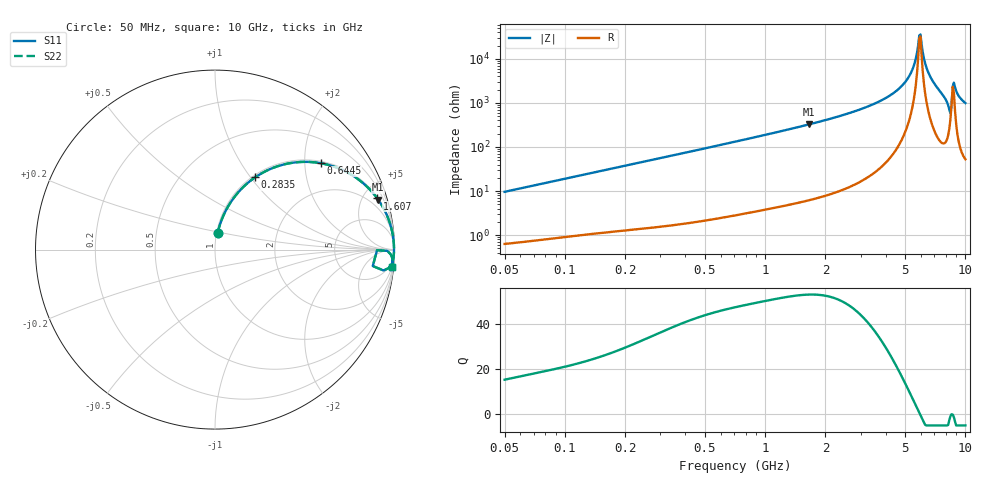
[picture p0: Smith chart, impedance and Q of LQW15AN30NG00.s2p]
!Murata Part Number: LQW15AN30NG00
!These Parameters are Measured in Series Mode Connection
!  o--[Z]--o
!Port1  Port2
!  o-------o
!Freq. Start=50[MHz] Stop=10[GHz], 401[Steps]
# Hz S RI R 50
!Freq.(Hz)	S 11(Real)	S 11(Imag)	S 21(Real)	S 21(Imag)	S 12(Real)	S 12(Imag)	S 22(Real)	S 22(Imag)
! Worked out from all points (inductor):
!   401 points, 50 MHz to 10 GHz, reference 50 ohm
!   read as one part in series: L = 30.3 nH near 51.34 MHz
!   highest Q = 52.9 at 1.651 GHz (marker M1), where L = 31.3 nH
!   self-resonance near 5.887 GHz
!   S11 on the Smith chart (normalised r, x): 50 MHz: 1.01, +0.19; 283.5 MHz: 1.03, +1.05; 644.5 MHz: 1.05, +2.40; 1.607 GHz: 1.12, +6.30; 10 GHz: 2, -20
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5e7  0.0151 0.0936  0.9849 -0.0936  0.9849 -0.0936  0.0151 0.0936
1.214486e8  0.0581 0.2131  0.9419 -0.2131  0.9419 -0.2131  0.0581 0.2131
2.835028e8  0.2239 0.4029  0.7761 -0.4029  0.7761 -0.4029  0.2239 0.4029
2.949953e8  0.2373 0.4117  0.7627 -0.4117  0.7627 -0.4117  0.2373 0.4117
6.444912e8  0.5879 0.4816  0.4121 -0.4816  0.4121 -0.4816  0.5879 0.4816
7.071068e8  0.6317 0.4719  0.3683 -0.4719  0.3683 -0.4719  0.6317 0.4719
1.607477e9  0.904 0.2852  0.096 -0.2852  0.096 -0.2852  0.904 0.2852
1.65063e9  0.909 0.2783  0.091 -0.2783  0.091 -0.2783  0.909 0.2783
1.717543e9  0.9161 0.2679  0.0839 -0.2679  0.0839 -0.2679  0.9161 0.2679
2.956399e9  0.9772 0.1383  0.0228 -0.1383  0.0228 -0.1383  0.9772 0.1383
4.171863e9  0.9927 0.0682  0.00726 -0.0682  0.00726 -0.0682  0.9927 0.0682
5.225452e9  0.9969 0.0249  0.00306 -0.0249  0.00306 -0.0249  0.9969 0.0249
5.583245e9  0.9974 0.012  0.0026 -0.012  0.0026 -0.012  0.9974 0.012
5.809576e9  0.9975 0.00413  0.0025 -0.00413  0.0025 -0.00413  0.9975 0.00413
5.965537e9  0.9975 -0.00118  0.00251 0.00118  0.00251 0.00118  0.9975 -0.00118
6.290134e9  0.9973 -0.0121  0.00275 0.0121  0.00275 0.0121  0.9973 -0.0121
6.54512e9  0.9969 -0.0205  0.00313 0.0205  0.00313 0.0205  0.9969 -0.0205
8.198065e9  0.9668 -0.1034  0.0332 0.1034  0.0332 0.1034  0.9668 -0.1034
8.307378e9  0.9391 -0.1163  0.0609 0.1163  0.0609 0.1163  0.9391 -0.1163
8.876195e9  0.9856 -0.041  0.0144 0.041  0.0144 0.041  0.9856 -0.041
9.359165e9  0.9888 -0.0726  0.0112 0.0726  0.0112 0.0726  0.9888 -0.0726
1e10  0.9849 -0.0984  0.0151 0.0984  0.0151 0.0984  0.9849 -0.0984
